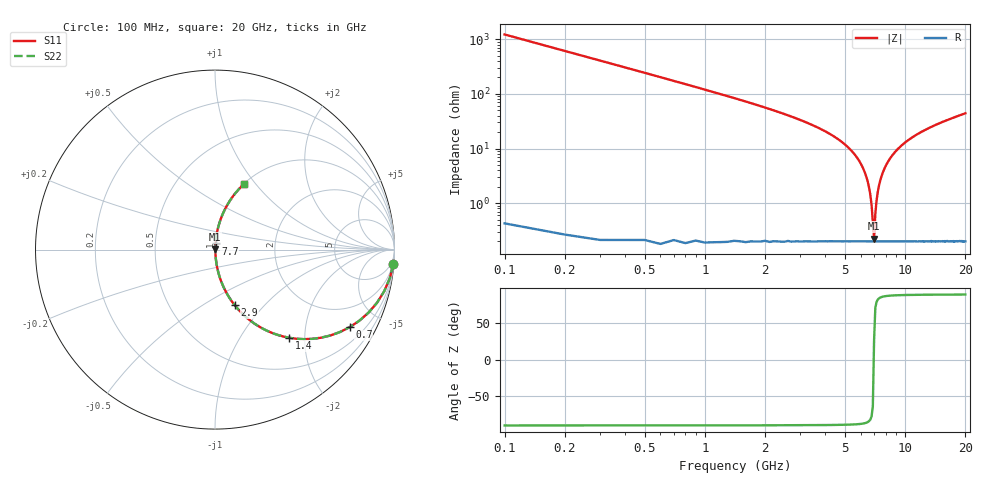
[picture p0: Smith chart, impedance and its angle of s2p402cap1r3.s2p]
! AVX Thin Film Operation		Date: April 2003
! Description: Accu-P® Series, Thin Film, SMD, RF Capacitor
! Part Number: 04023J1R3ABW
! 50 MHz  -  20 GHz
! Serial Measurements
# hz S db R 50
!	S11		S21		S12		S22
!	dB	Phase	dB	Phase	dB	Phase	dB	Phase
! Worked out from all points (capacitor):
!   200 points, 100 MHz to 20 GHz, reference 50 ohm
!   read as one part in series: C = 1.3 pF near 200 MHz
!   lowest |Z| = 225 mohm at 7 GHz (marker M1)
!   series resonance near 6.98 GHz, so ESL is about 400 pH
!   S11 on the Smith chart (normalised r, x): 100 MHz: 1, -24; 700 MHz: 1.00, -3.46; 1.4 GHz: 1.00, -1.68; 2.9 GHz: 1.00, -0.70; 7.7 GHz: 1.00, +0.07; 20 GHz: 1.00, +0.88
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1e8  -0.03 -4.7  -21.78 85.3  -21.78 85.3  -0.03 -4.7
2e8  -0.12 -9.3  -15.84 80.7  -15.84 80.7  -0.12 -9.3
3e8  -0.26 -13.8  -12.45 76.2  -12.45 76.2  -0.26 -13.8
7e8  -1.25 -30.0  -6.02 59.9  -6.02 59.9  -1.25 -30.0
1.4e9  -3.85 -49.9  -2.33 40.0  -2.33 40.0  -3.85 -49.9
2.1e9  -6.60 -61.9  -1.09 27.9  -1.09 27.9  -6.60 -61.9
2.9e9  -9.65 -70.5  -0.52 19.2  -0.52 19.2  -9.65 -70.5
3.5e9  -11.94 -74.9  -0.30 14.6  -0.30 14.6  -11.94 -74.9
5e9  -18.55 -82.2  -0.08 6.8  -0.08 6.8  -18.55 -82.2
5.9e9  -24.58 -84.7  -0.03 3.4  -0.03 3.4  -24.58 -84.7
6.5e9  -32.04 -84.0  -0.02 1.4  -0.02 1.4  -32.04 -84.0
6.8e9  -40.60 -77.1  -0.02 0.5  -0.02 0.5  -40.60 -77.1
7e9  -52.97 27.3  -0.02 -0.1  -0.02 -0.1  -52.97 27.3
7.1e9  -43.98 71.2  -0.02 -0.3  -0.02 -0.3  -43.98 71.2
7.2e9  -39.11 79.0  -0.02 -0.6  -0.02 -0.6  -39.11 79.0
7.4e9  -33.73 83.3  -0.02 -1.2  -0.02 -1.2  -33.73 83.3
7.7e9  -29.24 84.7  -0.02 -2.0  -0.02 -2.0  -29.24 84.7
8.6e9  -22.68 84.2  -0.04 -4.2  -0.04 -4.2  -22.68 84.2
1.01e10  -17.64 81.6  -0.09 -7.5  -0.09 -7.5  -17.64 81.6
1.34e10  -12.47 75.8  -0.27 -13.8  -0.27 -13.8  -12.47 75.8
1.67e10  -9.72 70.6  -0.51 -19.1  -0.51 -19.1  -9.72 70.6
2e10  -7.89 66.0  -0.79 -23.8  -0.79 -23.8  -7.89 66.0
